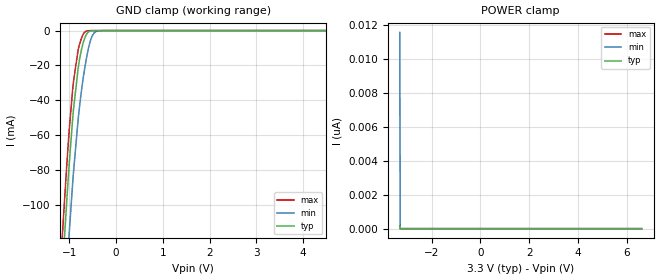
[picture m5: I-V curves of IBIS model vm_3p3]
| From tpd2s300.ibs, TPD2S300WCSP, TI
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|   VM_3p3 Model
[Model]   vm_3p3
Model_type   Input
Vinl = 0.99
Vinh = 2.31
|   typ   min   max
C_comp   15.2832pF   11.0063pF   19.7046pF
[Model spec]
|subparameter
Vinl   0.99   0.9897   0.9903
Vinh   2.31   2.3093   2.3107
| Where nom  PVT is Nominal Process, 3.3V, 27C
|   Fast PVT is Strong Process,  3.301V, -40C
|   Slow PVT is Weak Process,   3.299V, 125C
[Voltage Range]   3.3   3.299   3.301
[Temperature Range]   27   125   -40
[Power Clamp Reference]   3.3   3.299   3.301
[GND Clamp Reference]   0   0   0
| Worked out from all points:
|   GND clamp passes 1 mA (typ) near -0.60 V on its own axis
[GND Clamp]
|   Voltage   I(typ)   I(min)   I(max)
-3.3V     -1.248A    -1.347A    -1.203A
-1.171V   -147.9mA   -190.9mA   -126.3mA
-1.132V   -129.8mA   -172.2mA   -108.6mA
-1.063V   -99.63mA   -140.7mA   -79.12mA
-1.003V   -75.7mA    -115.3mA   -56.36mA
-914.1mV  -45.26mA   -81.33mA   -29.23mA
-815.1mV  -21.82mA   -51.21mA   -11.18mA
-735.9mV  -10.07mA   -33.06mA   -3.904mA
-646.8mV  -2.719mA   -17.4mA    -377.2uA
-537.9mV  -135uA     -4.709mA   -10.25uA
-399.3mV  -1.004uA   -226.2uA   0A
6.6V      0A         0A         0A
[POWER Clamp]
|   Voltage   I(typ)   I(min)   I(max)
-3.3V     180.3pA    11.59nA    149.9pA
-3.28V    0A         0A         0A
-3.27V    0A         0A         0A
6.6V      0A         0A         0A
